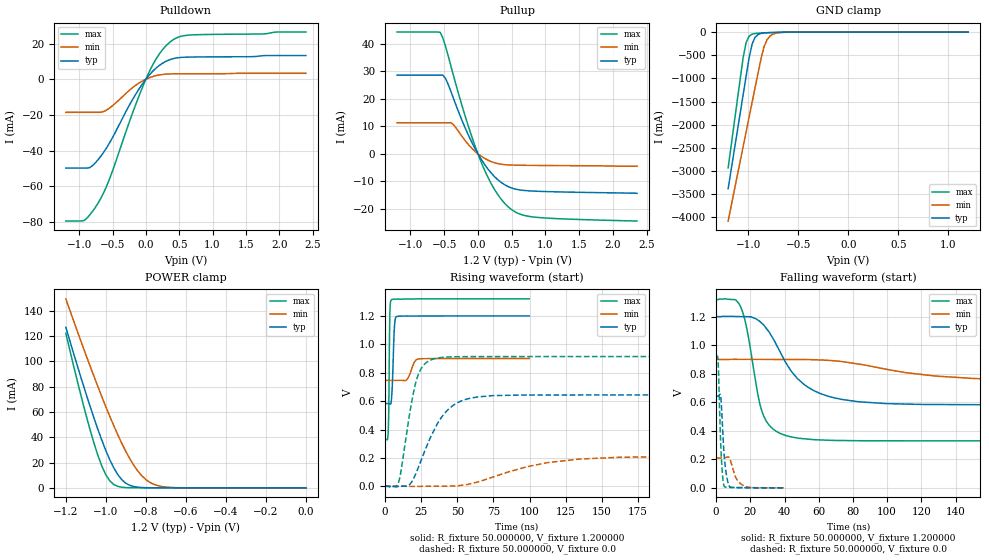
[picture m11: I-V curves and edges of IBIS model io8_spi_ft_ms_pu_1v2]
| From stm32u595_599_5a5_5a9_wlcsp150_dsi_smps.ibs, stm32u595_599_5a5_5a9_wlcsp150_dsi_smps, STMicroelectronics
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|   Model io8_spi_ft_ms_pu_1v2
[Model]  io8_spi_ft_ms_pu_1v2
Model_type I/O
Polarity   Non-Inverting
Enable   Active-Low
Vinl =   0.360000V
Vinh =   0.840000V
Vmeas =  0.600000V
Cref =   50.000000pF
Rref =   100.000000M
Vref =   0.0V
C_comp   3.132800pF   3.069700pF   3.178000pF
[Temperature Range]   25.000000   0.140000k   -40.000000
[Pullup Reference]   1.200000V   0.900000V   1.320000V
[Pulldown Reference]   0.0V   0.0V   0.0V
[POWER Clamp Reference]   1.200000V   0.900000V   1.320000V
[GND Clamp Reference]   0.0V   0.0V   0.0V
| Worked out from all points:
|   slope of the pulldown table from 0 to 0.18 V, typ, clamps not added: 25.4 ohm
|   slope of the pullup table from 0 to 0.18 V, typ, clamps not added: 27.8 ohm
|   GND clamp passes 1 mA (typ) near -0.51 V on its own axis
|   POWER clamp passes 1 mA (typ) near -0.86 V on its own axis
|   rising waveform, R_fixture 50.000000, V_fixture 1.200000: 20-80 % time 1.26ns typ, 3.37ns min, 604ps max; typ from 0.583 V to 1.2 V
|   rising waveform, R_fixture 50.000000, V_fixture 0.0: 20-80 % time 18.4ns typ, 45.6ns min, 9.08ns max; typ from 0 V to 0.643 V
|   falling waveform, R_fixture 50.000000, V_fixture 1.200000: 20-80 % time 21.9ns typ, 54.7ns min, 9.21ns max; typ from 1.2 V to 0.583 V
|   falling waveform, R_fixture 50.000000, V_fixture 0.0: 20-80 % time 2.21ns typ, 4.2ns min, 1.59ns max; typ from 0.643 V to 0 V
[Pulldown]
|Voltage   I(typ)   I(min)   I(max)
-1.2V     -49.85mA   -18.57mA   -79.56mA
-920mV    -49.85mA   -18.57mA   -79.19mA
-840mV    -49.59mA   -18.57mA   -76.08mA
-720mV    -45.32mA   -18.57mA   -69.73mA
-560mV    -36.71mA   -16.58mA   -57.44mA
-200mV    -11.43mA   -4.74mA    -19.03mA
0V        0A         0A         0A
160mV     6.476mA    2.075mA    11.78mA
360mV     10.99mA    2.989mA    20.81mA
480mV     12.07mA    3.053mA    23.52mA
640mV     12.42mA    3.074mA    24.76mA
2.4V      13.3mA     3.33mA     26.5mA
[Pullup]
|Voltage   I(typ)   I(min)   I(max)
-1.2V     28.64mA    11.31mA    44.33mA
-560mV    28.64mA    11.31mA    44.24mA
-480mV    27.41mA    11.31mA    39.11mA
-360mV    20.01mA    10.55mA    28.26mA
-160mV    7.809mA    3.931mA    11.44mA
40mV      -1.649mA   -721.3uA   -2.521mA
240mV     -8.14mA    -3.2mA     -12.72mA
360mV     -10.68mA   -3.85mA    -16.99mA
480mV     -12.27mA   -4.078mA   -19.94mA
640mV     -13.22mA   -4.169mA   -22.09mA
880mV     -13.63mA   -4.232mA   -23.13mA
2.36V     -14.4mA    -4.5mA     -24.46mA
[GND_clamp]
|Voltage   I(typ)   I(min)   I(max)
-1.2V     -3.379A    -4.076A    -2.932A
-1.05V    -1.35A     -2.47A     -550.7mA
-1.02V    -947.8mA   -2.149A    -221.5mA
-990mV    -552.4mA   -1.829A    -88.44mA
-960mV    -255.3mA   -1.51A     -44.87mA
-930mV    -111.8mA   -1.191A    -30.68mA
-870mV    -28.35mA   -564.6mA   -21.34mA
-840mV    -18.65mA   -309.5mA   -18.49mA
-810mV    -14.07mA   -161.6mA   -15.92mA
-780mV    -11.37mA   -83.33mA   -13.53mA
-600mV    -3.009mA   -4.321mA   -3.091mA
1.2V      0A         13.65nA    0A
[POWER_clamp]
|Voltage   I(typ)   I(min)   I(max)
-1.2V     127mA      149.4mA    122.2mA
-1.12V    84.98mA    114mA      70.29mA
-1.06V    55.52mA    88.42mA    35.69mA
-1.02V    37.64mA    72.04mA    17.19mA
-1V       29.52mA    64.13mA    10.33mA
-960mV    15.7mA     48.99mA    2.596mA
-900mV    3.636mA    28.77mA    207.8uA
-840mV    502.9uA    13.24mA    43.56uA
-800mV    129uA      6.535mA    43.56uA
-740mV    25.5uA     1.726mA    43.56uA
-620mV    25.17uA    82.33uA    36.07uA
0V        0A         17.36nA    0A
[Ramp]
| variable   typ   min   max
dV/dt_r  0.38569/18.35296n   0.12563/45.54480n   0.54818/9.06675n
dV/dt_f  0.37035/21.84693n   92.14800m/54.65019n 0.59404/9.19710n
R_load = 50.000000
[Rising Waveform]
R_fixture= 50.000000
V_fixture= 1.200000
V_fixture_min= 0.900000
V_fixture_max= 1.320000
|time   V(typ)   V(min)   V(max)
0s        582.7mV    746.1mV    330mV
2.202ns   582.8mV    746.1mV    379.7mV
2.603ns   582.7mV    746.1mV    525.4mV
3.403ns   580.1mV    746.1mV    1.226V
4.404ns   604.3mV    746.1mV    1.313V
6.406ns   1.101V     746.1mV    1.318V
7.808ns   1.194V     746.1mV    1.318V
15.02ns   1.199V     750.2mV    1.319V
22.82ns   1.199V     896.7mV    1.32V
99.7ns    1.2V       900mV      1.32V
[Rising Waveform]
R_fixture= 50.000000
V_fixture= 0.0
V_fixture_min= 0.0
V_fixture_max= 0.0
|time   V(typ)   V(min)   V(max)
0s        435.6uV    496.8uV    380.1uV
9.009ns   -1.15mV    495.3uV    17.25mV
16.82ns   11.59mV    -311uV     495.7mV
21.62ns   96.56mV    -613.8uV   743.2mV
25.23ns   189.9mV    -150.7uV   833.2mV
33.03ns   376.9mV    881.8uV    894.9mV
45.65ns   558.6mV    2.061mV    911.4mV
63.66ns   628.8mV    29.36mV    913.7mV
134.5ns   643.2mV    192mV      913.8mV
299.1ns   643.3mV    210mV      913.8mV
[Falling Waveform]
R_fixture= 50.000000
V_fixture= 1.200000
V_fixture_min= 0.900000
V_fixture_max= 1.320000
|time   V(typ)   V(min)   V(max)
0s        1.2V       900mV      1.32V
13.81ns   1.2V       900.7mV    1.281V
18.02ns   1.2V       900.6mV    1.111V
27.03ns   1.15V      900.5mV    528mV
32.43ns   1.063V     900.2mV    421.5mV
40.84ns   875.6mV    900mV      366.8mV
57.06ns   682.5mV    898.2mV    338mV
83.48ns   603.5mV    867.5mV    330.6mV
150.2ns   583.1mV    766.9mV    330mV
299.1ns   582.7mV    746.1mV    330mV
[Falling Waveform]
R_fixture= 50.000000
V_fixture= 0.0
V_fixture_min= 0.0
V_fixture_max= 0.0
|time   V(typ)   V(min)   V(max)
0s        643.3mV    210mV      913.8mV
1.201ns   642.8mV    210mV      873.4mV
2.643ns   645.5mV    210mV      315.4mV
3.684ns   440.3mV    209.8mV    98.03mV
4.725ns   222.8mV    209.9mV    10.83mV
6.326ns   69.75mV    215.8mV    4.298mV
8.168ns   5.899mV    198.9mV    3.125mV
11.85ns   2.102mV    63.99mV    2.792mV
16.66ns   1.646mV    11.94mV    1.59mV
39.88ns   435.6uV    496.8uV    380.1uV
